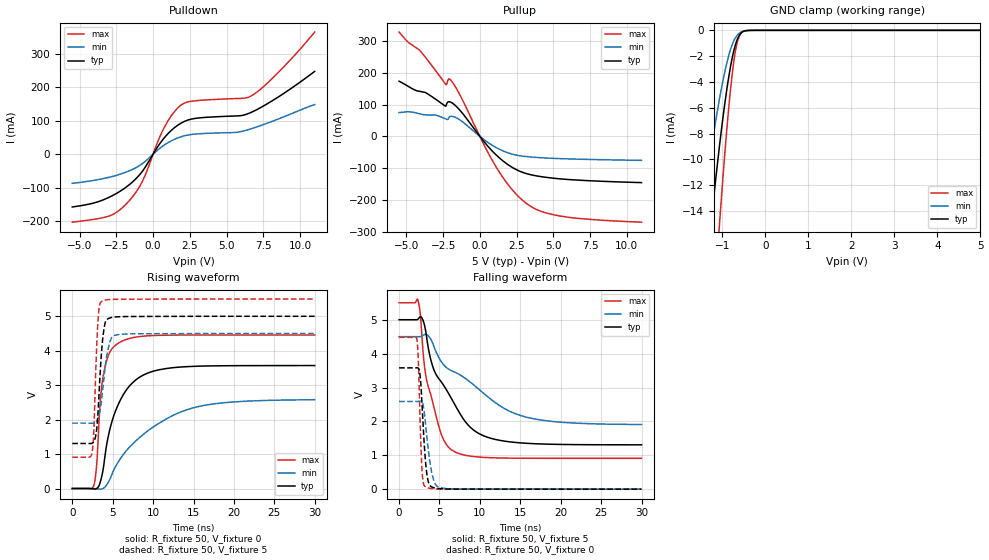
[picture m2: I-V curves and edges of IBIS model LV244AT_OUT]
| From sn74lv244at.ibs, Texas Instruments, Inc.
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[Model]   LV244AT_OUT
Model_type  3-state
Enable   Active-Low
Vref =   0
Rref =   1000
Cref =   50p
Vmeas =   1.5
| variable   typ   min   max
C_comp   4.11pF   3.11pF   4.82pF
| C_pullup   7.08pF   3.28pF   11.85pF
| C_pulldown   6.81pF   3.85pF   11.74pF
| C_tri-state   4.11pF   3.11pF   4.82pF
[Temperature Range]   40   100   -40
| Ambient temperature   25   85   -40
[Voltage range]   5   4.5   5.5
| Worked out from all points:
|   slope of the pulldown table from 0 to 0.75 V, typ, clamps not added: 15.5 ohm
|   slope of the pullup table from 0 to 0.75 V, typ, clamps not added: 18 ohm
|   GND clamp passes 1 mA (typ) near -0.69 V on its own axis
|   rising waveform, R_fixture 50, V_fixture 0: 20-80 % time 2.76ns typ, 6.89ns min, 1.01ns max; typ from 0 V to 3.57 V
|   falling waveform, R_fixture 50, V_fixture 5: 20-80 % time 4.48ns typ, 8ns min, 2.14ns max; typ from 5 V to 1.31 V
|   rising waveform, R_fixture 50, V_fixture 5: 20-80 % time 593ps typ, 831ps min, 419ps max; typ from 1.31 V to 5 V
|   falling waveform, R_fixture 50, V_fixture 0: 20-80 % time 553ps typ, 809ps min, 356ps max; typ from 3.58 V to 0 V
[GND Clamp]
| LV244AT_OUT
|   Voltage   I(typ)   I(min)   I(max)
-5.5V     -228mA     -149.7mA   -287mA
-1.54V    -24.85mA   -15.68mA   -39.41mA
-1.485V   -22.78mA   -14.34mA   -36.39mA
-1.26V    -14.88mA   -9.182mA   -24.47mA
-1.08V    -9.319mA   -5.552mA   -15.62mA
-1.055V   -8.61mA    -5.091mA   -14.46mA
-910mV    -4.881mA   -2.716mA   -8.194mA
-840mV    -3.372mA   -1.805mA   -5.572mA
-765mV    -2.035mA   -1.051mA   -3.212mA
-655mV    -716.1uA   -380.9uA   -950.6uA
-545mV    -149.8uA   -102.8uA   -148.9uA
5V        66.21nA    4.462nA    635.2nA
[Pulldown]
| LV244AT_OUT
|   Voltage   I(typ)   I(min)   I(max)
-5.5V     -157.8mA   -87.14mA   -203.3mA
-2.975V   -128.4mA   -68.75mA   -184.5mA
-1.725V   -94.85mA   -51.6mA    -144mA
-725mV    -50.87mA   -28.07mA   -81.03mA
335mV     23.73mA    13.24mA    39.13mA
835mV     52.74mA    29.57mA    85.85mA
1.865V    91.83mA    51.57mA    145.6mA
2.82V     106.7mA    60.04mA    159.5mA
5.62V     114.3mA    65.19mA    166.4mA
6.675V    125mA      76.05mA    174.2mA
8.565V    172.3mA    106.1mA    246.3mA
11V       247.6mA    148.4mA    365.1mA
[Pullup]
| LV244AT_OUT
|   Voltage   I(typ)   I(min)   I(max)
-5.5V     173.7mA    74.89mA    328.5mA
-4.9V     158.2mA    77.67mA    297.3mA
-4.045V   141.3mA    70.44mA    268.3mA
-2.31V    95.97mA    54.84mA    163.4mA
-2.115V   109.2mA    58.62mA    180.8mA
-1.885V   105.1mA    63.04mA    171.6mA
1.105V    -58.37mA   -35.22mA   -96.24mA
2.105V    -94.93mA   -54.59mA   -162.7mA
3.09V     -116.2mA   -63.24mA   -208.5mA
4.085V    -126.3mA   -66.98mA   -234.7mA
5.505V    -134mA     -70.14mA   -251.2mA
11V       -145.6mA   -75.58mA   -270.3mA
[Ramp]
| LV244AT_OUT
| variable   typ   min   max
dV/dt_r   2.15/2.76E-09   1.56/6.88E-09   2.68/1.01E-09
dV/dt_f   2.27/4.47E-09   1.60/8.01E-09   2.82/2.14E-09
R_load = 50
[Rising Waveform]
| LV244AT_OUT
R_fixture =   50
C_fixture =   0
L_fixture =   0
V_fixture =   0
V_fixture_min = 0
V_fixture_max = 0
|   Time   V(typ)   V(min)   V(max)
0s        1.266nV    819pV      2.497nV
2.685ns   -13.22mV   -851.3uV   99.95mV
3.01ns    -1.568mV   -8.029mV   665mV
3.45ns    176.9mV    -18.75mV   2.486V
3.845ns   593.9mV    5.126mV    3.288V
4.615ns   1.684V     247.8mV    3.943V
5.725ns   2.458V     782.3mV    4.222V
8.675ns   3.28V      1.55V      4.42V
14.32ns   3.54V      2.298V     4.456V
29.99ns   3.569V     2.579V     4.457V
[Falling Waveform]
| LV244AT_OUT
R_fixture =   50
C_fixture =   0
L_fixture =   0
V_fixture =   5
V_fixture_min = 4.5
V_fixture_max = 5.5
|   Time   V(typ)   V(min)   V(max)
0s        5V         4.5V       5.5V
2.325ns   5.014V     4.499V     5.589V
2.925ns   5.005V     4.535V     4.181V
3.47ns    4.383V     4.551V     3.15V
5.245ns   3.158V     3.754V     1.606V
6.615ns   2.615V     3.481V     1.14V
8.885ns   1.811V     3.143V     972.7mV
11.84ns   1.471V     2.564V     924.1mV
17.5ns    1.334V     2.042V     911.1mV
29.99ns   1.308V     1.906V     910.3mV
[Rising Waveform]
| LV244AT_OUT
R_fixture =   50
C_fixture =   0
L_fixture =   0
V_fixture =   5
V_fixture_min = 4.5
V_fixture_max = 5.5
|   Time   V(typ)   V(min)   V(max)
0s        1.308V     1.898V     910.3mV
2.445ns   1.314V     1.896V     1.044V
2.65ns    1.357V     1.898V     1.587V
2.965ns   1.62V      1.943V     3.797V
3.17ns    2.155V     2.028V     4.827V
3.615ns   3.943V     2.549V     5.427V
4.115ns   4.841V     3.615V     5.472V
4.665ns   4.952V     4.26V      5.487V
5.24ns    4.979V     4.446V     5.492V
29.99ns   5V         4.5V       5.5V
[Falling Waveform]
| LV244AT_OUT
R_fixture =   50
C_fixture =   0
L_fixture =   0
V_fixture =   0
V_fixture_min = 0
V_fixture_max = 0
|   Time   V(typ)   V(min)   V(max)
0s        3.579V     2.588V     4.481V
2.205ns   3.582V     2.588V     4.415V
2.37ns    3.572V     2.59V      3.856V
2.61ns    3.337V     2.595V     1.96V
2.815ns   2.607V     2.571V     657.7mV
3.205ns   1.013V     2.078V     77.6mV
3.56ns    277.3mV    1.272V     39.31mV
4.05ns    65.83mV    477.2mV    15.64mV
4.985ns   14.81mV    55.16mV    3.888mV
29.99ns   2.071uV    18.68uV    15.75nV
